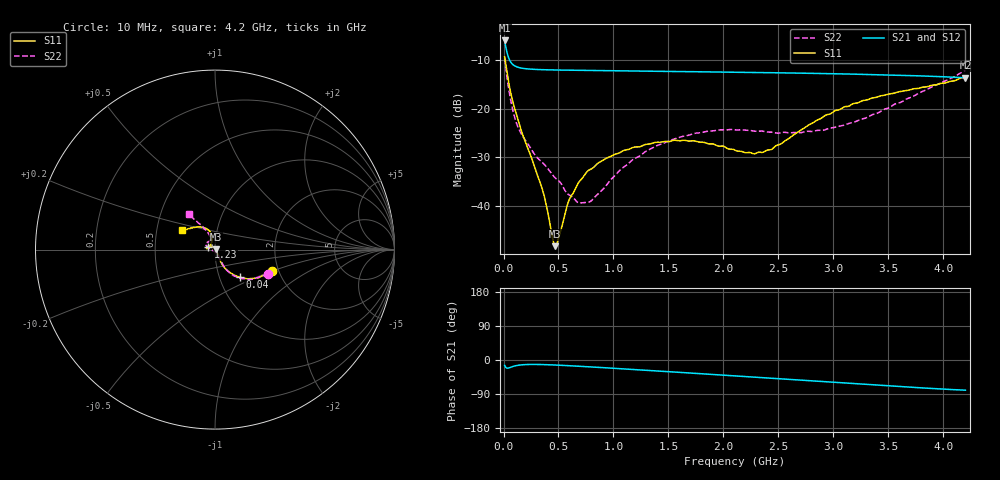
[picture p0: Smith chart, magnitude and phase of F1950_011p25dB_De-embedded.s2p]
! Integrated Device Technology
! Corporate Headquarters
! 6024 Silver Creek Valley Road
! San Jose, CA 95138  USA
! Phone:  1-408-284-8200
! Toll Free:  1-800-223-1366
! Webpage:  http://www.idt.com/
! Timing and RF Division
! 515 Groton Road, Suite 102
! Westford, MA 01886-6024
! Device:  F1950
! Description: 7-bit 0.25 dB Digital Step Attenuator
! Frequency:  150.0 -  4000.00 MHz
! Package:  4x4 mm Thin QFN Plastic Package: 24 pin
! Ports:  2 RF, 12 DC
!  Pin  1  = D0
!  Pin  2  = VDD
!  Pin  3  = Vmode
!  Pin  4  = GND
!  Pin  5  = RF1  =  Port 1
!  Pin  6  = GND
!  Pin  7  = GND
!  Pin  8  = GND
!  Pin  9  = GND
!  Pin 10  = GND
!  Pin 11  = GND
!  Pin 12  = GND
!  Pin 13  = GND
!  Pin 14  = RF2  =  Port 2
!  Pin 15  = GND
!  Pin 16  = LE
!  Pin 17  = CLK
!  Pin 18  = DATE
!  Pin 19  = D6
!  Pin 20  = D5
!  Pin 21  = D4
!  Pin 22  = D3
!  Pin 23  = D2
!  Pin 24  = D1
! State:  45
! Atten State:  11.25 dB
! Voltage:  +5.00 Volts
! Current:  Not Measured mA
! Data:  The device was measured on a the F195X evaluation board which has
!  individual transmission lines to the RF pins.  Data was collected
!  using a calibrated network analyzer.  The evaluation board was
!  de-embedded using a TRL calibration technique.
!  The reference plane is the edge of the package pin.
! Misc:  Board 2019
!  Action Tracker AT0250
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# GHz S dB R 50
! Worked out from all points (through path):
!   420 points, 10 MHz to 4.2 GHz, reference 50 ohm
!   highest |S21| = -6.05 dB at 10 MHz (marker M1); lowest = -13.7 dB at 4.2 GHz (marker M2)
!   group delay of S21, straight-line fit = 48.7 ps
!   lowest |S11| = -48.2 dB at 470 MHz (marker M3), VSWR 1.01, Z = 50.3 + j0.201 ohm
!   |S11| at or under -10 dB: 14.32 MHz to end of sweep
!   |S22| runs from -39.3 to -9.7 dB; largest |S21 - S12| = 0.00032
!   S11 on the Smith chart (normalised r, x): 10 MHz: 1.85, -0.49; 40 MHz: 1.25, -0.40; 1.23 GHz: 0.93, +0.03; 4.2 GHz: 0.68, +0.15
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0.01  -9.38 -20.1  -6.05 -14.1  -6.04 -14.1  -9.74 -24.7
0.04  -13.72 -48.3  -9.18 -21.6  -9.18 -21.6  -14.97 -54.6
0.09  -19.05 -62.5  -11.07 -16.7  -11.07 -16.7  -20.84 -62.2
0.15  -23.68 -64.5  -11.65 -13.2  -11.65 -13.2  -24.68 -63.6
0.35  -36.29 -47.2  -12.03 -12.0  -12.03 -12.0  -30.95 -66.6
0.45  -46.95 -0.9  -12.08 -13.0  -12.08 -13.0  -33.71 -70.2
0.47  -48.17 30.8  -12.09 -13.2  -12.09 -13.3  -34.18 -73.1
0.5  -46.59 73.0  -12.10 -13.6  -12.10 -13.6  -34.75 -75.5
0.6  -38.50 114.5  -12.14 -15.1  -12.14 -15.1  -37.74 -90.4
0.71  -34.40 126.1  -12.17 -16.8  -12.17 -16.9  -39.27 -117.1
0.79  -32.44 131.7  -12.19 -18.2  -12.19 -18.2  -39.01 -141.1
0.92  -30.37 140.0  -12.23 -20.4  -12.23 -20.4  -36.14 -169.5
1.23  -27.84 156.9  -12.32 -25.9  -12.32 -25.9  -29.81 168.3
1.41  -26.89 164.8  -12.36 -29.1  -12.36 -29.2  -27.44 162.6
1.73  -26.60 172.7  -12.45 -35.0  -12.44 -35.0  -25.11 154.5
2.11  -28.56 163.3  -12.55 -42.2  -12.55 -42.2  -24.37 144.4
2.28  -29.26 144.8  -12.60 -45.3  -12.60 -45.4  -24.61 138.5
2.43  -28.42 126.4  -12.65 -48.1  -12.65 -48.1  -24.80 132.8
2.81  -22.96 103.7  -12.78 -55.4  -12.78 -55.4  -24.67 116.0
3.1  -19.63 106.4  -12.90 -60.9  -12.90 -61.0  -23.38 110.7
3.51  -16.98 118.6  -13.11 -68.5  -13.11 -68.5  -19.79 113.1
4.2  -13.52 149.4  -13.70 -79.6  -13.69 -79.7  -12.20 126.9
